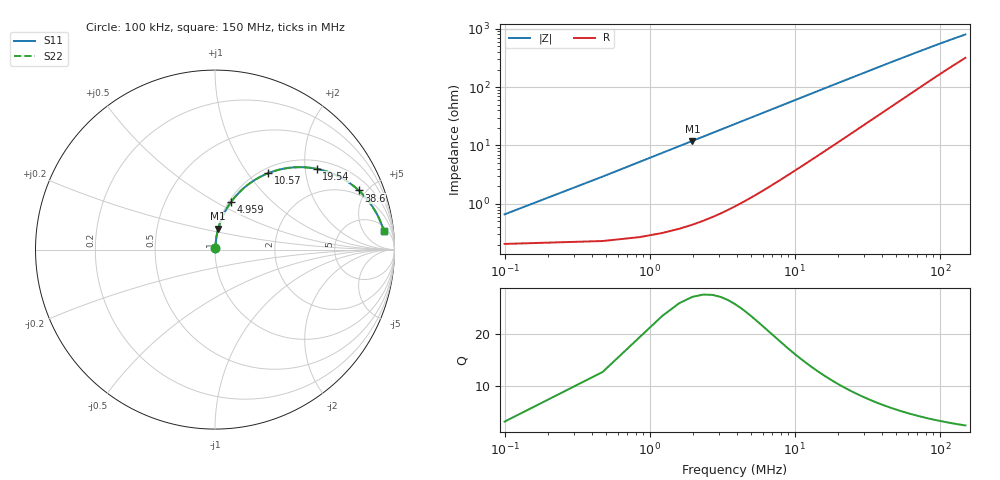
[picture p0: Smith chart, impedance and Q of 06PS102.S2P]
! Coilcraft 0603PS-102 Power Chip Inductor
! 19 February 2003
# MHZ S MA R 50
!Freq  MagS11  AngS11  MagS21  AngS21  MagS12  AngS12  MagS22  AngS22
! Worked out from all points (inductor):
!   403 points, 100 kHz to 150 MHz, reference 50 ohm
!   read as one part in series: L = 971 nH near 847.6 kHz
!   highest Q = 26.6 at 1.969 MHz (marker M1), where L = 966 nH
!   S11 on the Smith chart (normalised r, x): 100 kHz: 1.00, +0.01; 4.959 MHz: 1.03, +0.60; 10.57 MHz: 1.08, +1.26; 19.54 MHz: 1.22, +2.30; 38.6 MHz: 1.68, +4.45; 150 MHz: 7, +15
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0.1  0.006595 71.5  0.9979 -0.4  0.9979 -0.4  0.006595 71.5
0.4738  0.02923 83.8  0.9973 -1.7  0.9973 -1.7  0.02923 83.8
1.2214  0.07415 83.3  0.9941 -4.2  0.9941 -4.2  0.07415 83.3
1.5952  0.09631 82.3  0.9917 -5.5  0.9917 -5.5  0.09631 82.3
1.969  0.1183 81.1  0.9887 -6.8  0.9887 -6.8  0.1183 81.1
2.3428  0.14 79.9  0.9851 -8.0  0.9851 -8.0  0.14 79.9
3.0904  0.1825 77.4  0.9765 -10.5  0.9765 -10.5  0.1825 77.4
3.838  0.2238 74.9  0.966 -12.9  0.966 -12.9  0.2238 74.9
4.9594  0.2829 71.2  0.9472 -16.4  0.9472 -16.4  0.2829 71.2
6.0808  0.3383 67.6  0.9254 -19.7  0.9254 -19.7  0.3383 67.6
7.576  0.4057 63.1  0.893 -23.9  0.893 -23.9  0.4057 63.1
10.5664  0.5189 55.1  0.8223 -31.2  0.8223 -31.2  0.5189 55.1
14.3044  0.6245 47.0  0.7341 -38.5  0.7341 -38.5  0.6245 47.0
19.5376  0.723 38.5  0.6255 -46.0  0.6255 -46.0  0.723 38.5
25.1446  0.7884 31.9  0.5326 -51.6  0.5326 -51.6  0.7884 31.9
31.1254  0.8321 26.9  0.4563 -55.6  0.4563 -55.6  0.8321 26.9
38.6014  0.8661 22.4  0.3852 -58.9  0.3852 -58.9  0.8661 22.4
50.1892  0.8961 17.7  0.3091 -61.7  0.3091 -61.7  0.8961 17.7
75.2338  0.9246 12.1  0.2168 -63.7  0.2168 -63.7  0.9246 12.1
100.2784  0.9365 9.2  0.1681 -63.3  0.1681 -63.3  0.9365 9.2
125.323  0.9429 7.4  0.1384 -62.0  0.1384 -62.0  0.9429 7.4
150  0.9468 6.3  0.1187 -60.3  0.1187 -60.3  0.9468 6.3
